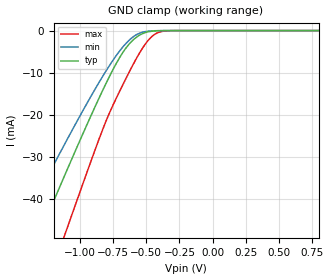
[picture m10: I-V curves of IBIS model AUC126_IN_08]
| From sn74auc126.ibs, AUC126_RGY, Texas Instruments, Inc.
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[Model]   AUC126_IN_08
Model_type  Input
Vinl=0
Vinh=0.8
| variable   typ   min   max
C_comp   2.45pF   2.11pF   2.75pF
[Temperature Range]   40   100   -40
| Ambient temperature   25   85   -40
[Voltage range]   0.8   0.8   0.8
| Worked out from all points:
|   GND clamp passes 1 mA (typ) near -0.55 V on its own axis
[GND Clamp]
| AUC126_IN_08
|   Voltage   I(typ)   I(min)   I(max)
-3.6V     -222.3mA   -186mA     -267.4mA
-1.455V   -59.64mA   -47.59mA   -78.96mA
-1.32V    -49.54mA   -39.29mA   -66.93mA
-1.275V   -46.2mA    -36.55mA   -62.91mA
-1.115V   -34.42mA   -26.97mA   -48.63mA
-1.08V    -31.87mA   -24.92mA   -45.5mA
-825mV    -13.98mA   -10.69mA   -23.23mA
-695mV    -6.113mA   -4.618mA   -14.06mA
-580mV    -1.724mA   -1.091mA   -6.949mA
-450mV    -123.7uA   -58.22uA   -1.212mA
-315mV    -2.431uA   -1.512uA   -21.15uA
800mV     96.17pA    179pA      76.88pA
